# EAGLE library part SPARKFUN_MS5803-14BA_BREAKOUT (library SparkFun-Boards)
SparkFun MSP5803-14BA Breakout I2C compatible pressure sensor breakout SparkFun Products: SparkFun MSP5803-14BA Breakout
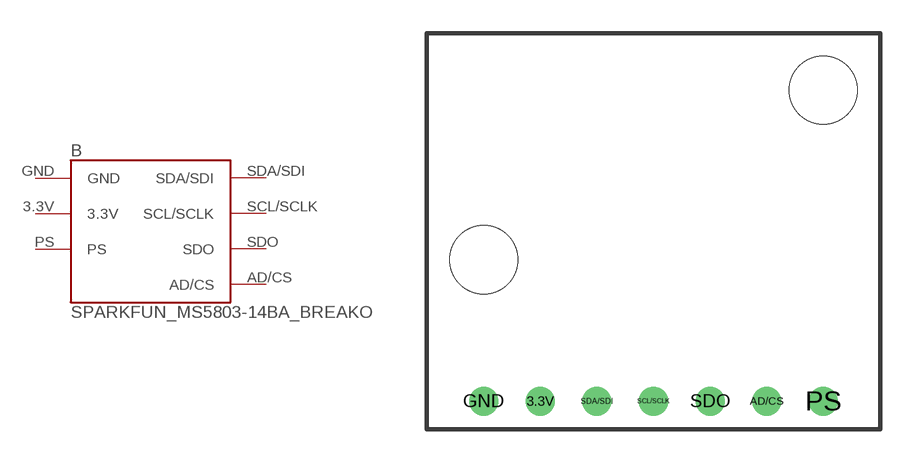
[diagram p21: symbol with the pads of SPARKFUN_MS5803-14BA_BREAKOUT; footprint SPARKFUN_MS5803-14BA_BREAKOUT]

Designator prefix B

## SPARKFUN_MS5803-14BA_BREAKOUT (SF_ID: SEN-12909; VALUE: Pressure Sensor)  [SPARKFUN_MS5803-14BA_BREAKOUT]
3.3V  3.3V
AD/CS  AD/CS
GND  GND
PS  PS
SCL/SCLK  SCL/SCLK
SDA/SDI  SDA/SDI
SDO  SDO

## Footprint SPARKFUN_MS5803-14BA_BREAKOUT (pad centres in mm)
SparkFun MS5803-14BA Breakout Specifications: Pin count:7 Pin pitch: 0.1" Area: 0.8x0.7" Example device(s): SPARKFUN_MS5803-14BA_BREAKOUT
drill 0.8: 3.3V 5.08,1.27; AD/CS 15.24,1.27; GND 2.54,1.27; PS 17.78,1.27; SCL/SCLK 10.16,1.27; SDA/SDI 7.62,1.27; SDO 12.7,1.27
hole 3.048 at 2.54,7.62
hole 3.048 at 17.78,15.24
